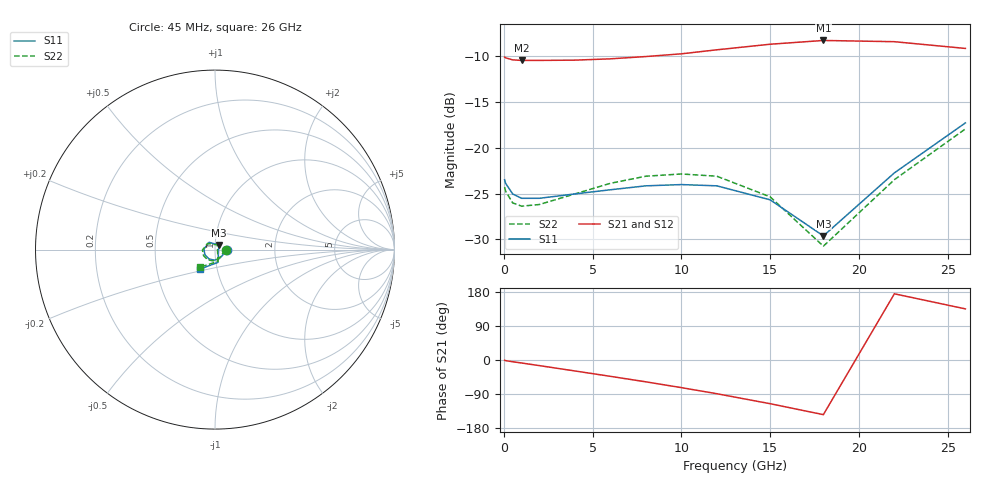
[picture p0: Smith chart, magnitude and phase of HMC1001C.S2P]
! HMMC-1001
! Typical s-parameters at 10dB attenuation setting, TA = 25 C
# ghz s ma r 50
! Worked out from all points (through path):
!   14 points, 45 MHz to 26 GHz, reference 50 ohm
!   highest |S21| = -8.25 dB at 18 GHz (marker M1); lowest = -10.4 dB at 1 GHz (marker M2)
!   lowest |S11| = -29.6 dB at 18 GHz (marker M3), VSWR 1.07, Z = 52.1 + j2.63 ohm
!   |S11| at or under -10 dB: start of sweep to end of sweep
!   |S22| runs from -30.8 to -17.9 dB; largest |S21 - S12| = 0.0055
0.045  0.067 -2.8  0.314 -0.6  0.313 -0.8  0.061 -3.7
0.1  0.064 -6.5  0.311 -1.7  0.31 -1.7  0.058 -8.3
0.5  0.056 -12.8  0.303 -4.6  0.303 -4.4  0.05 -14.3
1  0.053 -18.8  0.301 -7.9  0.301 -7.8  0.048 -22.8
2  0.053 -33.9  0.301 -14.8  0.3 -14.8  0.049 -40.7
4  0.056 -64.5  0.302 -28.9  0.303 -28.9  0.056 -73.5
6  0.059 -94.1  0.307 -43.1  0.308 -43.1  0.064 -101.1
8  0.062 -123.4  0.316 -57.6  0.316 -57.8  0.07 -127.3
10  0.063 -153.0  0.327 -72.9  0.328 -72.9  0.072 -152.7
12  0.062 177.8  0.344 -89.0  0.343 -88.9  0.07 -178.0
15  0.052 128.8  0.369 -115.3  0.367 -115.2  0.054 140.4
18  0.033 49.7  0.387 -144.2  0.386 -144.5  0.029 64.2
22  0.073 -77.1  0.381 174.7  0.383 174.7  0.067 -75.2
26  0.137 -127.7  0.35 134.9  0.35 134.0  0.127 -129.8
